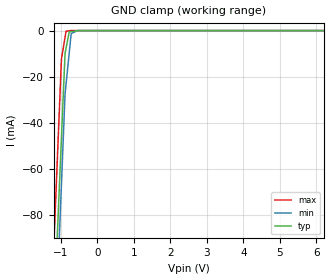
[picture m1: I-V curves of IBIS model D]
|Texas Instruments Incorporated
|2,4-channel protection solution for super-speed (6 GBPS) USB 3.0 interface
| Marketing part#   Voltage Range(Digital)   Package-type   #pin
|TPD2EUSB30ADRTR   4.5V to 5.5V   SOT   3
|TPD2EUSB30DRTR   4.5V to 5.5V   SOT   3
[IBIS Ver]   4.1
[File name]   tpd2eusb30a.ibs
[File Rev]   1.0
[Date]   05/12/2011
[Source]   Texas Instruments Incorporated.
   Analog-eLab, HPA
   12500 TI Blvd
   Dallas, TX -75243
   For Support e-mail: elab_ibis@list.ti.com
[Notes]   Revision History:
   1.0: 05/12/2011
   - Initial version of the model
   - Initial Model generated from simulations.
   - Model not matched to measurements
   - ccomp values are based on PVT conditions although listed
   in numerical order.
[Disclaimer]
 This product is designed as an aid for customers of Texas Instruments.
 No warranties, either expressed or implied, with respect to this third
 party software (if any) or with respect to its fitness for any
 particular purpose is claimed by Texas Instruments or the author. The
 software (if any) is provided solely on an "as is" basis. The entire
 risk as to its quality and performance is with the customer
[Copyright] (C) Copyright 2011 Texas Instruments Incorporated.
   All rights reserved.
|   tpd2eusb30a
[Component]   tpd2eusb30a
[Manufacturer] TI
[Package]   | 3 pin  package
| variable   typ   min   max
R_pkg   0.2308   0.2247   0.2425
L_pkg   1.1348nH   1.1090nH   1.1726nH
C_pkg   0.0986pF   0.0921pF   0.1050pF
|-------------------------PIN------------------------------------------------
[Pin] signal_name  model_name   R_pin   L_pin   C_pin
1   D+   D   0.2247   1.1090nH   0.0921pF
2   D-   D   0.2253   1.1230nH   0.0986pF
3   GND   GND   0.2425   1.1726nH   0.1050pF
| Models and submodels in the file (1): D (Input)
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|   D
[Model]   D
Model_type   Input
Vinl = 0.3
Vinh = 0.9
|   typ   min   max
C_comp   0.6pF   0.6pF   0.6pF
[Voltage Range]   5   4.5   5.5
[Temperature Range]   40   100   -40
[Power Clamp Reference]   5   4.5   5.5
[GND Clamp Reference]   -0   -0   -0
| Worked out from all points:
|   GND clamp passes 1 mA (typ) near -0.78 V on its own axis
[GND Clamp]
|   Voltage   I(typ)   I(min)   I(max)
-5V       -1.965A    -1.986A    -1.941A
-1.185V   -122mA     -147.3mA   -90.57mA
-983mV    -46.69mA   -66.88mA   -12.34mA
-884.6mV  -9.946mA   -27.64mA   -2.92mA
-856.9mV  -7.677mA   -23.31mA   -268.2uA
-770.5mV  -605.4uA   -9.805mA   -86.45uA
-716.1mV  -461.1uA   -1.292mA   -2.457uA
-547.6mV  -14.58uA   -39.87uA   0A
10V       0A         0A         0A
